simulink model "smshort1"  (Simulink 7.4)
settings: Solver=ode45  StartTime=0.0  StopTime=10  MaxStep=1e-3  RelTol=1e-4  AbsTol=1e-4
InitFcn:
  | smshort2data
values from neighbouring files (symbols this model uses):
  Bm = 0.10    (= 0.1)    [IMabc2.m]    (also in imabcparam.m = 0.01; IMabcrun0.m = 0.01; IMabcrun1.m = 0.001; IMcur0.m = 1e-06)
  H = 0.60    (= 0.6)    [IMabc2.m]    (also in IMcur0.m = 0.3; imdef0vec.m = 0.3; imdef1vec.m = 0.3; imdef2vec.m = 0.3)
  Ra = .95    (= 0.95)    [altwdgs.m]    (also in Ccurverun.m = 0.018)
  Tl = Tl2    [calc0.m]
  V = [Vas 0 0].'    [Actac.m]    (also in acttrcalc1.m = str2num(get(h,'string')); im3d.m = eval(get(hVs,'String')); IMabc2.m = [vas vbs vcs 0 0 0]'; IMabcf0.m = [vas vbs vcs 0 0 0]')
  wo = 2*pi*freq0    [calc0.m]    (also in IMabc2.m = 376.991118431; imabcparam.m = 376.991118431; IMabcrun0.m = 376.991118431; IMabcrun1.m = 376.991118431)
undefined symbols (not defined in the file or in its folder): Lal, Lfl, Lkdl, Lkql, Lmd, Lmq, Rf, Rkd, Rkq, vf0
libraries: simulink x1

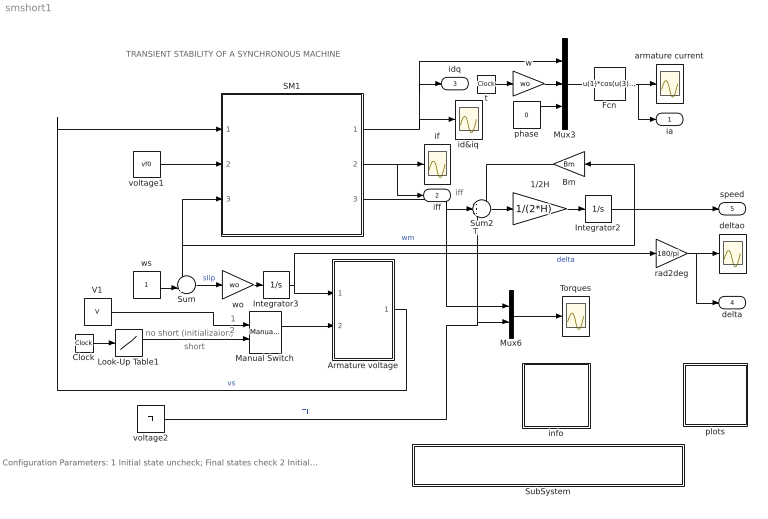
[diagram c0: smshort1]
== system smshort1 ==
  note: Tl
  note: TRANSIENT STABILITY OF A SYNCHRONOUS MACHINE
  note: iff
  note: short
  note: no short (initializaion)
  note: 1
  note: 2
  note: Configuration Parameters: 1 Initial state uncheck; Final states check 2 Initial state check; Final states uncheck
  1/2H : Gain  Gain=1/(2*H)  ParameterDataType=sfix(16)  ParameterScaling=2^0  OutDataType=sfix(16)  OutScaling=2^0
  Armature voltage : Subsystem
  Bm : Gain  Gain=Bm  ParameterDataType=sfix(16)  ParameterScaling=2^0  OutDataType=sfix(16)  OutScaling=2^0
  Clock : Clock
  Fcn : Fcn  Expr=u(1)*cos(u(3)+u(4))+u(2)*sin(u(3)+u(4))
  Integrator2 : Integrator  InitialCondition=1
  Integrator3 : Integrator  InitialCondition=-pi/6
  Look-Up Table1 : Lookup  InputValues=[0 0.5 0.5 0.6 0.6 5]  Table=[V V 0 0 V V]  OutDataType=sfix(16)  OutScaling=2^0
  Manual Switch : simulink/Signal Routing/Manual Switch  SystemSampleTime=-1  sw=0  action=0  varsize=off
  Mux3 : Mux  Inputs=3
  Mux6 : Mux  Inputs=2
  SM1 : Subsystem
  SubSystem : Subsystem
  Sum : Sum  Inputs=-+|  OutDataType=sfix(16)  OutScaling=2^0
  Sum2 : Sum  Inputs=-+-  OutDataType=sfix(16)  OutScaling=2^0
  Torques : Scope
  V1 : Constant  Value=V  OutDataType=sfix(16)  OutScaling=2^0
  armature current : Scope
  deltao : Scope
  id&iq : Scope
  if : Scope
  info : Subsystem
  phase : Constant  Value=0  OutDataType=sfix(16)  OutScaling=2^0
  plots : Subsystem
  rad2deg : Gain  Gain=180/pi  ParameterDataType=sfix(16)  ParameterScaling=2^0  OutDataType=sfix(16)  OutScaling=2^0
  t : Clock
  voltage1 : Constant  Value=vf0  OutDataType=sfix(16)  OutScaling=2^0
  voltage2 : Constant  Value=Tl  OutDataType=sfix(16)  OutScaling=2^0
  w : Gain  Gain=wo  ParameterDataType=sfix(16)  ParameterScaling=2^0  OutDataType=sfix(16)  OutScaling=2^0
  wo : Gain  Gain=wo  ParameterDataType=sfix(16)  ParameterScaling=2^0  OutDataType=sfix(16)  OutScaling=2^0
  ws : Constant  OutDataType=sfix(16)  OutScaling=2^0
  ia : Outport
  iff : Outport  Port=2
  idq : Outport  Port=3
  delta : Outport  Port=4
  speed : Outport  Port=5
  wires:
  voltage1/1 -> SM1/2(vf)
  1/2H/1 -> Integrator2/1
  Sum2/1 -> 1/2H/1
  Bm/1 -> Sum2/1
  ws/1 -> Sum/2
  Sum/1 -> wo/1  "slip"
  Armature voltage/1(vs) -> SM1/1(vs)  "vs"
  wo/1 -> Integrator3/1
  Integrator3/1 -> Armature voltage/1(delta), rad2deg/1  "delta"
  Clock/1 -> Look-Up Table1/1
  Integrator2/1 -> Bm/1, Sum/1, SM1/3(wm), speed/1  "wm"
  voltage2/1 -> Mux6/2, Sum2/3  "Tl"
  w/1 -> Mux3/2
  phase/1 -> Mux3/3
  Mux3/1 -> Fcn/1
  t/1 -> w/1
  Fcn/1 -> armature current/1, ia/1
  SM1/2(if) -> if/1, iff/1
  SM1/3(Te) -> Sum2/2, Mux6/1
  SM1/1(ia) -> id&iq/1, Mux3/1, idq/1
  Manual Switch/1 -> Armature voltage/2(Vt)
  Look-Up Table1/1 -> Manual Switch/2
  V1/1 -> Manual Switch/1
  Mux6/1 -> Torques/1
  rad2deg/1 -> deltao/1, delta/1

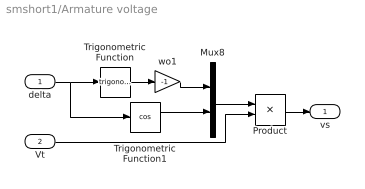
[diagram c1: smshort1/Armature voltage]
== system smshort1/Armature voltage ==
  delta : Inport  OutDataType=sfix(16)  OutScaling=2^0
  Vt : Inport  Port=2  OutDataType=sfix(16)  OutScaling=2^0
  Mux8 : Mux  Inputs=2
  Product : Product  OutDataType=sfix(16)  OutScaling=2^0
  Trigonometric Function : Trigonometry
  Trigonometric Function1 : Trigonometry  Operator=cos
  wo1 : Gain  Gain=-1  ParameterDataType=sfix(16)  ParameterScaling=2^0  OutDataType=sfix(16)  OutScaling=2^0
  vs : Outport
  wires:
  delta/1 -> Trigonometric Function/1, Trigonometric Function1/1
  Trigonometric Function/1 -> wo1/1
  Mux8/1 -> Product/1
  wo1/1 -> Mux8/1
  Trigonometric Function1/1 -> Mux8/2
  Product/1 -> vs/1
  Vt/1 -> Product/2

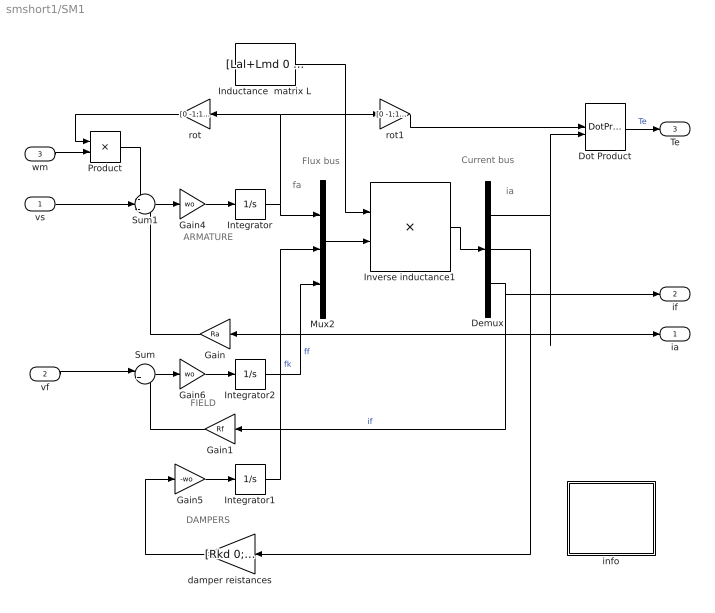
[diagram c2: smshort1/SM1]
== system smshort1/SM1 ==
  note: DAMPERS
  note: ARMATURE
  note: fa
  note: ia
  note: FIELD
  note: Flux bus
  note: Current bus
  vs : Inport  OutDataType=sfix(16)  OutScaling=2^0
  vf : Inport  Port=2  OutDataType=sfix(16)  OutScaling=2^0
  wm : Inport  Port=3  OutDataType=sfix(16)  OutScaling=2^0
  Demux : Demux  Outputs=3
  Dot Product : DotProduct  OutDataType=fixdt(1, 16)  OutScaling=2^-10
  Gain : Gain  Gain=Ra  ParameterDataType=sfix(16)  ParameterScaling=2^0  OutDataType=sfix(16)  OutScaling=2^0
  Gain1 : Gain  Gain=Rf  ParameterDataType=sfix(16)  ParameterScaling=2^0  OutDataType=sfix(16)  OutScaling=2^0
  Gain4 : Gain  Gain=wo  ParameterDataType=sfix(16)  ParameterScaling=2^0  OutDataType=sfix(16)  OutScaling=2^0
  Gain5 : Gain  Gain=-wo  ParameterDataType=sfix(16)  ParameterScaling=2^0  OutDataType=sfix(16)  OutScaling=2^0
  Gain6 : Gain  Gain=wo  ParameterDataType=sfix(16)  ParameterScaling=2^0  OutDataType=sfix(16)  OutScaling=2^0
  Inductance  matrix L : Constant  Value=[Lal+Lmd 0 Lmd 0 Lmd;0 Lal+Lmq 0 Lmq 0;Lmd 0 Lmd+Lkdl 0 Lmd;0 Lmq 0 Lmq+Lkql 0;Lmd 0 Lmd 0 Lmd+Lfl]  VectorParams1D=off  OutDataType=fixdt(1, 16)  OutScaling=2^0
  Integrator : Integrator
  Integrator1 : Integrator
  Integrator2 : Integrator  InitialCondition=2
  Inverse inductance1 : Product  Inputs=/*  Multiplication=Matrix(*)  OutDataType=sfix(16)  OutScaling=2^0
  Mux2 : Mux  Inputs=3
  Product : Product  OutDataType=sfix(16)  OutScaling=2^0
  Sum : Sum  Inputs=|+-  OutDataType=sfix(16)  OutScaling=2^0
  Sum1 : Sum  Inputs=-+-  OutDataType=sfix(16)  OutScaling=2^0
  damper reistances : Gain  Gain=[Rkd 0;0 Rkq]  Multiplication=Matrix(K*u)  ParameterDataType=sfix(16)  ParameterScaling=2^0  OutDataType=sfix(16)  OutScaling=2^0
  info : Subsystem
  rot : Gain  Gain=[0 -1;1 0]  Multiplication=Matrix(K*u)  ParameterDataType=sfix(16)  ParameterScaling=2^0  OutDataType=sfix(16)  OutScaling=2^0
  rot1 : Gain  Gain=[0 -1;1 0]  Multiplication=Matrix(K*u)  ParameterDataType=sfix(16)  ParameterScaling=2^0  OutDataType=sfix(16)  OutScaling=2^0
  ia : Outport
  if : Outport  Port=2
  Te : Outport  Port=3
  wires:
  Product/1 -> Sum1/1
  rot/1 -> Product/1
  wm/1 -> Product/2
  Gain5/1 -> Integrator1/1
  damper reistances/1 -> Gain5/1
  Integrator/1 -> Mux2/1, rot/1, rot1/1
  Sum1/1 -> Gain4/1
  Gain4/1 -> Integrator/1
  vs/1 -> Sum1/2
  Gain/1 -> Sum1/3
  Gain6/1 -> Integrator2/1
  Sum/1 -> Gain6/1
  vf/1 -> Sum/1
  Gain1/1 -> Sum/2
  rot1/1 -> Dot Product/1
  Demux/1 -> Gain/1, ia/1, Dot Product/2
  Dot Product/1 -> Te/1  "Te"
  Integrator1/1 -> Mux2/2  "fk"
  Integrator2/1 -> Mux2/3  "ff"
  Demux/2 -> damper reistances/1
  Demux/3 -> if/1, Gain1/1  "if"
  Mux2/1 -> Inverse inductance1/2
  Inverse inductance1/1 -> Demux/1
  Inductance  matrix L/1 -> Inverse inductance1/1

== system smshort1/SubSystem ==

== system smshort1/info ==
  note: Transient stability of a synchronous machine
  note: To establish the running operating point prior to a short, set the manual switch in the up position 1 and the corresponding configuration parameters as described in bottom left block. To initiate the short conditions, go to position 2 and modify the configuration parameters.

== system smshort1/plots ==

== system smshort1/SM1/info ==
  note: Synchronous machine transients under shortcircuit
  note: This demonstration illustrates the dynamics of a synchronous generator, initially at no load, following a three-phase short circuit at the terminals.
